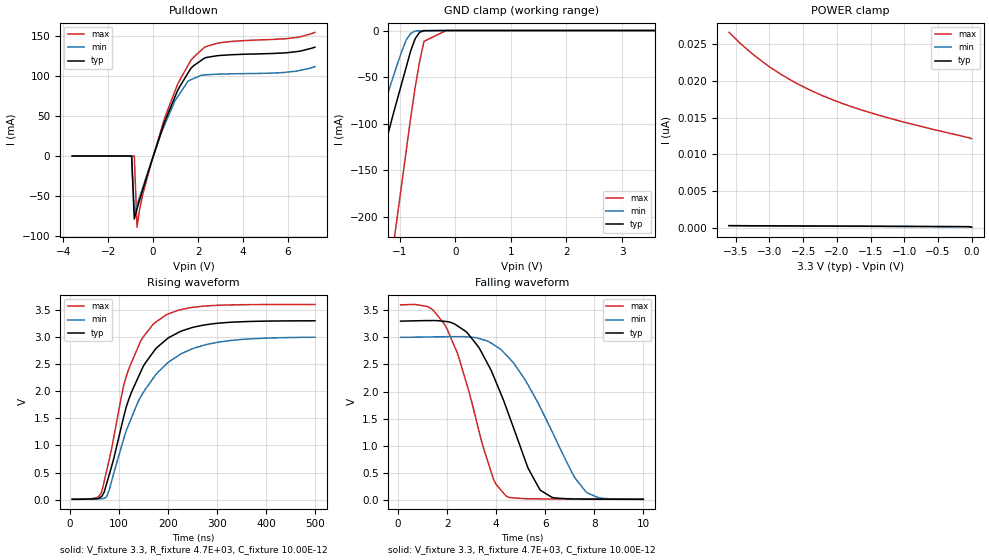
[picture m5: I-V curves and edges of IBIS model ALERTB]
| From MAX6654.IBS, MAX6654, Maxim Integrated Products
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|   ALERTB Output
[Model]   ALERTB
|Signals   ALERTB
Model_type   Open_drain
Polarity   Inverting
Vmeas = 1.65V
C_comp   1.532E-12   1.281E-12   1.784E-12
[Temperature Range]   25   -55   125
[Voltage Range]   3.30V   3.00V   3.60V
[Pullup Reference]   3.30V   3.00V   3.60V
[Pulldown Reference]   0.00V   0.00V   0.00V
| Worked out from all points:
|   slope of the pulldown table from 0 to 0.495 V, typ, clamps not added: 11.8 ohm
|   GND clamp passes 1 mA (typ) near -0.60 V on its own axis
|   rising waveform, V_fixture 3.3, R_fixture 4.7E+03, C_fixture 10.00E-12: 20-80 % time 76.9ns typ, 91.9ns min, 62.4ns max; typ from 0.008 V to 3.3 V
|   falling waveform, V_fixture 3.3, R_fixture 4.7E+03, C_fixture 10.00E-12: 20-80 % time 1.73ns typ, 2.08ns min, 1.39ns max; typ from 3.3 V to 0.012 V
[Pulldown]
| Note that the [Pulldown] voltage table is referenced to Gnd.
|V(V)   I(typ)   I(min)   I(max)
-3.6V     0A         0A         0A
-960mV    0A         0A         0A
-840mV    -78.85mA   -71.3mA    0A
-720mV    -66.21mA   -61.09mA   -89.05mA
-480mV    -43.68mA   -40.7mA    -50.21mA
480mV     40.38mA    36.9mA     44.83mA
960mV     73.4mA     68.65mA    80.53mA
1.56V     104.3mA    94.13mA    113.9mA
1.8V      113mA      96.95mA    123.6mA
2.28V     122.5mA    101.4mA    135.9mA
2.88V     125.6mA    102.4mA    141.3mA
7.2V      136.2mA    111.8mA    154.8mA
[POWER_clamp]
| Note that the [POWER_clamp] voltage table is referenced to Vcc
| and is calculated using Vtable=Vcc - Vmeasured.
|V(V)   I(typ)   I(min)   I(max)
-3.6V     331.2pA    324.5pA    26.58nA
-3.44V    324.7pA    318.2pA    25.15nA
-3.24V    316.7pA    310.2pA    23.56nA
-3V       307.1pA    300.7pA    21.91nA
-2.84V    300.6pA    294.4pA    20.94nA
-2.64V    292.7pA    286.5pA    19.87nA
-2.28V    278.3pA    272.4pA    18.25nA
-1.8V     259.4pA    253.7pA    16.54nA
-1.36V    242.1pA    236.8pA    15.28nA
-880mV    223.4pA    218.4pA    14.1nA
-40mV     191.3pA    187.2pA    12.27nA
0V        138.8pA    126pA      12.14nA
[GND_clamp]
| Note that the [GND_clamp] voltage table is referenced to Gnd.
|V(V)   I(typ)   I(min)   I(max)
-3.6V     -699.8mA   -531.2mA   -1.424A
-2V       -303.4mA   -218.7mA   -649.9mA
-1.92V    -283.7mA   -203.2mA   -611.5mA
-1.68V    -225mA     -156.9mA   -497mA
-1.6V     -205.5mA   -141.4mA   -458.8mA
-1.12V    -91mA      -50.58mA   -234.6mA
-1.04V    -73.69mA   -36.11mA   -199.3mA
-880mV    -39.05mA   -10.06mA   -128.8mA
-720mV    -8.739mA   -458.7uA   -61mA
-560mV    -270uA     -1.531uA   -11.53mA
-160mV    -22.18pA   66.18pA    -1.324uA
3.6V      276.6pA    114pA      12.41nA
[Ramp]
|variable   typ   min   max
dV/dt_r   3.30/7.685E-08   3.00/9.225E-08   3.60/6.247E-08
dV/dt_f   3.30/1.738E-09   3.00/2.086E-09   3.60/1.396E-09
R_load = 4.7E+03
[Rising Waveform]
V_fixture = 3.3
V_fixture_min = 3.0
V_fixture_max = 3.6
R_fixture = 4.7E+03
L_fixture = 0
C_fixture = 10.00E-12
|Time   V(typ)   V(min)   V(max)
5ns       7.71mV     6.815mV    8.288mV
50ns      15.77mV    11.53mV    27.03mV
65ns      60.59mV    18.27mV    141.3mV
80ns      449.2mV    170.2mV    723.7mV
115ns     1.709V     1.272V     2.269V
145ns     2.365V     1.903V     2.935V
175ns     2.781V     2.303V     3.273V
225ns     3.1V       2.68V      3.502V
280ns     3.229V     2.864V     3.573V
500ns     3.299V     2.995V     3.599V
[Falling Waveform]
V_fixture = 3.3
V_fixture_min = 3.0
V_fixture_max = 3.6
R_fixture = 4.7E+03
L_fixture = 0
C_fixture = 10.00E-12
|Time   V(typ)   V(min)   V(max)
100ps     3.3V       3V         3.599V
1.2ns     3.309V     3.007V     3.567V
1.9ns     3.295V     3.011V     3.236V
2.5ns     3.187V     3.013V     2.59V
3.3ns     2.809V     2.979V     1.266V
3.9ns     2.276V     2.863V     367.8mV
4.4ns     1.713V     2.677V     73.69mV
5.8ns     178.5mV    1.704V     19.76mV
7.7ns     16.61mV    133.4mV    14.49mV
10ns      12.27mV    12.96mV    11.57mV
